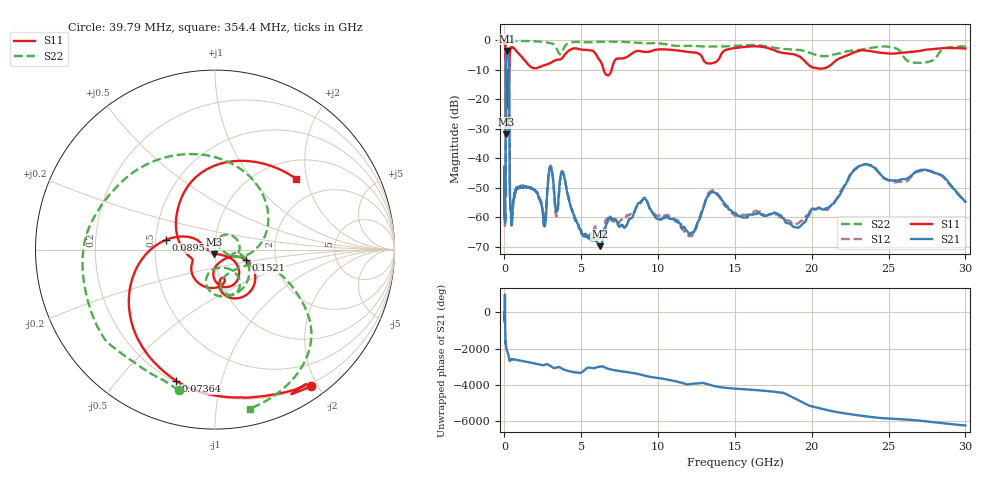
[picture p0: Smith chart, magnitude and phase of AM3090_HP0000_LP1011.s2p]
! Date/Time: Thu, Feb 28, 2019 1:53 PM
! Network Analyzer: Agilent Technologies E8364B Rev: A.07.50.67
! Sweep from 0.010 to 30.000 GHz, 1601 Points, Sweep Type: LOG
! Power Supply: 5.022 V, 0.002 A
# Hz S DB R 50
!freq MagS11 AngS11 MagS21 AngS21 MagS12 AngS12 MagS22 AngS22
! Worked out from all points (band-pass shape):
!   1601 points, 10 MHz to 30 GHz, reference 50 ohm
!   highest |S21| = -3.69 dB at 150.6 MHz (marker M1); lowest = -69.9 dB at 6.202 GHz (marker M2)
!   |S21| within 3 dB of the highest: 99.65 MHz to 283.9 MHz (184.2 MHz wide, 96.1 % of centre)
!   lowest |S11| = -32.0 dB at 97.94 MHz (marker M3), VSWR 1.05, Z = 49.3 - j2.41 ohm
!   |S11| at or under -10 dB: 88.91 MHz to 314.5 MHz (225.6 MHz wide, 112 % of centre); 6.455 GHz to 6.979 GHz (524.3 MHz wide, 7.81 % of centre)
!   |S22| runs from -31.1 to -0.2 dB; largest |S21 - S12| = 0.013
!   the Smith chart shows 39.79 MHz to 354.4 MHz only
!   S11 on the Smith chart (normalised r, x): 39.79 MHz: 0.17, -1.91; 73.64 MHz: 0.21, -0.73; 89.51 MHz: 0.57, +0.07; 152.1 MHz: 1.41, -0.17; 354.4 MHz: 1.40, +1.73
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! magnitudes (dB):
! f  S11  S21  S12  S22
! 10 MHz  -0.2  -43.0  -48.0  -0.7
! 38.04 MHz  -0.5  -59.9  -59.0  -1.7
! 39.79 MHz  -0.6  -61.6  -59.4  -1.9
! 73.64 MHz  -2.4  -48.2  -47.0  -4.3
! 89.51 MHz  -11.1  -15.0  -15.0  -11.5
! 97.94 MHz  -32.0  -7.3  -7.2  -30.1
! 113.8 MHz  -13.4  -4.8  -4.8  -18.7
! 144.7 MHz  -19.8  -3.7  -3.7  -19.3
! 150.6 MHz  -15.5  -3.7  -3.7  -17.3
! 152.1 MHz  -14.7  -3.7  -3.7  -16.7
! 288.7 MHz  -16.3  -7.4  -7.3  -15.4
! 354.4 MHz  -4.4  -52.1  -52.3  -0.8
! 550.5 MHz  -2.6  -56.2  -56.9  -0.3
! 2.084 GHz  -9.6  -51.6  -51.6  -0.5
! 2.61 GHz  -8.6  -63.1  -60.9  -0.7
! 2.958 GHz  -7.9  -43.2  -42.8  -1.0
! 3.385 GHz  -6.7  -58.3  -59.6  -2.7
! 3.798 GHz  -5.9  -44.9  -44.6  -3.5
! 6.202 GHz  -6.8  -69.9  -67.4  -0.6
! 7.926 GHz  -5.9  -62.8  -59.9  -0.7
! 23.48 GHz  -3.5  -42.1  -42.0  -3.0
! 30 GHz  -2.9  -54.8  -55.0  -2.2
